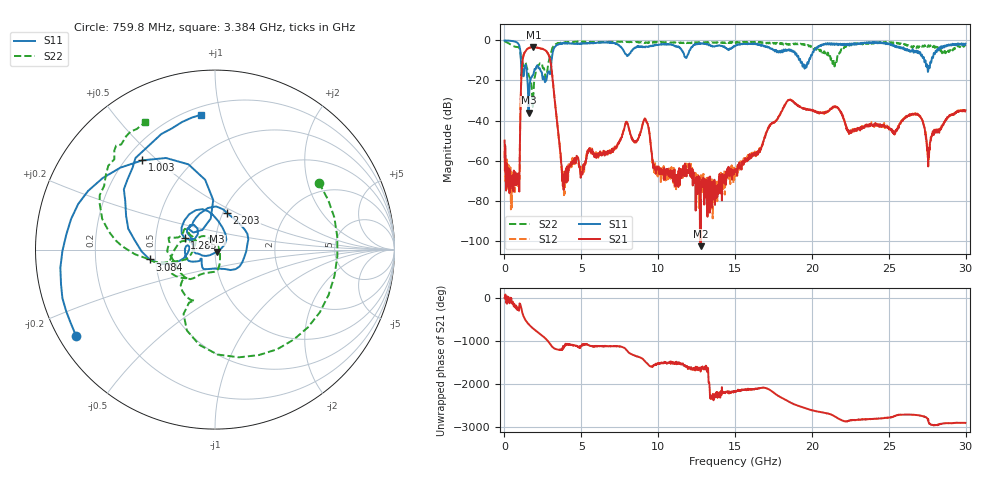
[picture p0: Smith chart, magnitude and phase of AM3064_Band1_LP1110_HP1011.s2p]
# Hz S DB R 50.0
!freq dBS11 angS11 dBS21 angS21 dBS12 angS12 dBS22 angS22
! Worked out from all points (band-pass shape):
!   1600 points, 10 MHz to 29.98 GHz, reference 50 ohm
!   highest |S21| = -3.34 dB at 1.884 GHz (marker M1); lowest = -102.7 dB at 12.76 GHz (marker M2)
!   |S21| within 3 dB of the highest: 1.293 GHz to 2.811 GHz (1.519 GHz wide, 74 % of centre)
!   lowest |S11| = -36.1 dB at 1.566 GHz (marker M3), VSWR 1.03, Z = 51.1 - j1.15 ohm
!   |S11| at or under -10 dB: 1.071 GHz to 3.064 GHz (1.992 GHz wide, 96.4 % of centre); 19.24 GHz to 19.8 GHz (562.2 MHz wide, 2.88 % of centre); 27.38 GHz to 27.78 GHz (405.2 MHz wide, 1.47 % of centre)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
!   |S22| runs from -32.9 to -0.4 dB; largest |S21 - S12| = 0.011
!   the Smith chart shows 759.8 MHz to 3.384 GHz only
!   S11 on the Smith chart (normalised r, x): 759.8 MHz: 0.05, -0.28; 1.003 GHz: 0.26, +0.45; 1.285 GHz: 0.71, +0.09; 2.203 GHz: 1.05, +0.45; 3.084 GHz: 0.46, -0.06; 3.384 GHz: 0.25, +0.87
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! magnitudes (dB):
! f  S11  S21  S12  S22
! 10 MHz  -0.1  -50.0  -55.5  -0.4
! 234.9 MHz  -0.1  -71.3  -65.3  -1.3
! 759.8 MHz  -0.8  -72.3  -68.1  -3.2
! 1.003 GHz  -3.9  -51.7  -51.8  -4.7
! 1.285 GHz  -14.9  -6.5  -6.4  -12.6
! 1.566 GHz  -36.1  -3.9  -3.9  -16.9
! 1.884 GHz  -16.9  -3.3  -3.4  -26.9
! 2.203 GHz  -13.4  -3.7  -3.7  -12.6
! 3.084 GHz  -8.7  -15.9  -15.7  -4.6
! 3.384 GHz  -2.4  -38.0  -37.9  -1.8
! 3.871 GHz  -1.4  -69.3  -77.2  -1.1
! 5.015 GHz  -1.6  -65.7  -64.9  -0.7
! 9.157 GHz  -3.5  -39.2  -39.1  -1.1
! 10 GHz  -2.2  -63.7  -64.0  -0.9
! 12.76 GHz  -1.7  -102.7  -70.5  -1.0
! 15 GHz  -2.9  -64.1  -65.0  -1.3
! 18.44 GHz  -5.0  -30.0  -30.0  -1.9
! 19.99 GHz  -7.4  -34.8  -34.8  -3.1
! 25 GHz  -1.5  -43.7  -44.0  -1.2
! 26.87 GHz  -6.3  -37.2  -37.3  -3.0
! 27.6 GHz  -12.7  -58.3  -59.2  -2.6
! 29.98 GHz  -1.6  -34.8  -35.1  -2.9
